| Texas Instruments Incorporated
| CDCLVP1102 1:2 Differential Buffer with one Clock Input
| CDCLVP1204 2:4 Differential Buffer with Selectable Clock Inputs
| CDCLVP1208 Low Jitter 8 Output LVPECL Buffer with Selectable Input
| CDCLVP1212 Low Jitter 12 Output LVPECL Buffer with Selectable Input
| CDCLVP1216 2:16 Differential LVPECL Buffer, High Performance Clock Buffer
| CDCLVP2102 Low Jitter Dual 1:2 LVPECL Buffer
| CDCLVP2104 Low Jitter Dual 1:4 LVPECL Buffer
| CDCLVP2106 Low Jitter Dual 1:6 LVPECL Buffer
| CDCLVP2108 1:8,16 LVPECL Output, no SEL pin,High Performance Clock Buffer
| Marketing part#   Voltage Range   Package-type   #pins/pkg drawing
| CDCLVP1102RGTR   2.375V - 3.6V   QFN   16-pin RGT
| CDCLVP1102RGTT   2.375V - 3.6V   QFN   16-pin RGT
| CDCLVP2102RGTR   2.375V - 3.6V   QFN   16-pin RGT
| CDCLVP2102RGTT   2.375V - 3.6V   QFN   16-pin RGT
| CDCLVP1204RGTR   2.375V - 3.6V   QFN   16-pin RGT
| CDCLVP1204RGTT   2.375V - 3.6V   QFN   16-pin RGT
| CDCLVP1216RGZR   2.375V - 3.6V   QFN   48-pin RGZ
| CDCLVP1216RGZT   2.375V - 3.6V   QFN   48-pin RGZ
| CDCLVP2108RGZR   2.375V - 3.6V   QFN   48-pin RGZ
| CDCLVP2108RGZT   2.375V - 3.6V   QFN   48-pin RGZ
| CDCLVP1212RHAR   2.375V - 3.6V   QFN   40-pin RHA
| CDCLVP1212RHAT   2.375V - 3.6V   QFN   40-pin RHA
| CDCLVP2106RHAR   2.375V - 3.6V   QFN   40-pin RHA
| CDCLVP2106RHAT   2.375V - 3.6V   QFN   40-pin RHA
| CDCLVP1208RHDR   2.375V - 3.6V   QFN   28-pin RHD
| CDCLVP1208RHDT   2.375V - 3.6V   QFN   28-pin RHD
| CDCLVP2104RHDR   2.375V - 3.6V   QFN   28-pin RHD
| CDCLVP2104RHDT   2.375V - 3.6V   QFN   28-pin RHD
[IBIS ver]   4.1
[File name]   cdclvpx.ibs
[File Rev]   1.3
[Date]   09/30/2013
[Source]
| Texas Instruments Incorporated.
| Analog-eLab Design Center, HPA
| 12500 TI Blvd
| Dallas, TX -75243
[Notes]   Revision History
| Rev 1.0: 06/03/2009
| - Initial model generated from Spectre simulations
| - Initial version of the model not matched to
|   measurements
| - Warnings related to VAC_REF clamp characterisitics
|   can be ignored, as they represent true buffer characteristics
| - Initial IBIS file named cdclvp1102.ibs
| Rev 1.1: 07/29/2009
| - File name changed from cdclvp1102.ibs to cdclvpx.ibs
| - Added package models for CDCLVP2102,CDCLVP1204,CDCLVP1216,CDCLVP2108,
|   CDCLVP1212, CDCLVP2106, CDCLVP1208, and CDCLVP2104. All these
|   parts share same set of I/O buffers.
| Rev 1.2: 08/20/2013
| - Added models for 2.5V corner.
| Rev 1.3: 09/30/2013
| - Modified pecl models at 3.3V and 2.5V corners.
|*  EXCEPTION:   *
|*  - For model input_2p5 and sel_in_2p5, there will be a leakage   *
|*   current in the POWER clamp I-V Table because of the transistor   *
|*   XQQ0 connected to the pad.   *
|*  - For model vac_ref_2p5, there will be a leakage current in the   *
|*   GROUND and POWER clamp I-V Table because of the voltage source   *
|*   connected  to the pad.   *
|*  - For model pecl_*, there will be a leakage current in the GROUND   *
|*   clamp I-V Table because of the BJT Q6<1:20>(NPN4T_3V_LC_P25L5)   *
|*   connected to the pad.   *
[Disclaimer]
| This model is designed as an aid for customers of Texas Instruments.
| TI and its licensors and suppliers make no warranties, either expressed
| or implied, with respect to this  model, including the warranties of
| merchantability or fitness for a particular purpose. The model is
| provided solely on an "as is" basis. The entire risk as to its quality
| and performance is with the customer.
[Copyright] (C)Copyright 2013 Texas Instruments Incorporated.
   All rights reserved.
|   Component CDCLVP1102RGT
[Component]   CDCLVP1102RGT
[Manufacturer]  Texas Instruments Incorporated
[Package]   |16-pin QFN RGT package
|   typ   min   max
R_pkg   0.2442   0.2257   0.2626
L_pkg   1.1009nH   1.0046nH   1.1974nH
C_pkg   0.1103pF   0.1081pF   0.1124pF
[Pin] signal_name  model_name   R_pin   L_pin   C_pin
   1   GND   GND   0.12037   0.82216nH   0.12472pF
   2   NC   NC   0.00244   0.06008nH   0.03612pF
   3   NC   NC   0.00244   0.06008nH   0.03612pF
   4   NC   NC   0.00244   0.06216nH   0.03162pF
   5   VCC   POWER   0.12566   0.86112nH   0.13739pF
   6   INP0   INPUT   0.22876   1.02355nH   0.11116pF
   7   INN0   INPUT   0.23258   1.04274nH   0.11153pF
   8   VAC_REF   VAC_REF   0.26260   1.19735nH   0.11242pF
   9   OUTP0   PECL_OUT   0.25027   1.13306nH   0.10811pF
   10   OUTN0   PECL_OUT   0.22571   1.00464nH   0.10867pF
   11   OUTP1   PECL_OUT   0.22940   1.02114nH   0.11008pF
   12   OUTN1   PECL_OUT   0.25984   1.17646nH   0.11074pF
   13   NC   NC   0.00244   0.06216nH   0.03162pF
   14   NC   NC   0.00244   0.06008nH   0.03612pF
   15   NC   NC   0.00244   0.06008nH   0.03612pF
   16   GND   GND   0.12148   0.82689nH   0.12554pF
[Diff_Pin]  inv_pin  vdiff   tdelay_typ  tdelay_min  tdelay_max
| The '+' pin is   Diff_pin,   the '-' pin is the   Inv_pin
| Receiver Pins  |  Receiver Vth = +/-200mV
6   7   0.8V   0ns   0ns   0ns
| LVPECL Driver Pins
9   10   0.5V   0ns   0ns   0ns
11   12   0.5V   0ns   0ns   0ns
|   Component CDCLVP2102RGT
[Component]   CDCLVP2102RGT
[Manufacturer]  Texas Instruments Incorporated
[Package]   |16-pin QFN RGT package
|   typ   min   max
R_pkg   0.2458   0.2257   0.2658
L_pkg   1.1055nH   1.0046nH   1.2064nH
C_pkg   0.1092pF   0.1051pF   0.1132pF
[Pin] signal_name  model_name   R_pin   L_pin   C_pin
   1   GND   GND   0.12037   0.82216nH   0.12819pF
   2   NC   NC   0.00244   0.06008nH   0.03612pF
   3   INP1   INPUT   0.22606   1.00656nH   0.10507pF
   4   INN1   INPUT   0.25236   1.14386nH   0.10913pF
   5   VCC   POWER   0.08325   0.79299nH   0.15518pF
   6   INP0   INPUT   0.22876   1.02355nH   0.11162pF
   7   INN0   INPUT   0.23258   1.04274nH   0.11159pF
   8   VAC_REF   VAC_REF   0.26260   1.19735nH   0.11246pF
   9   OUTP0   PECL_OUT   0.25027   1.13306nH   0.10814pF
   10   OUTN0   PECL_OUT   0.22571   1.00464nH   0.10870pF
   11   OUTP1   PECL_OUT   0.22940   1.02114nH   0.11016pF
   12   OUTN1   PECL_OUT   0.25984   1.17646nH   0.11123pF
   13   OUTP2   PECL_OUT   0.26581   1.20636nH   0.11324pF
   14   OUTN2   PECL_OUT   0.23400   1.04124nH   0.11179pF
   15   OUTP3   PECL_OUT   0.22794   1.01049nH   0.10931pF
   16   OUTN3   PECL_OUT   0.25004   1.12526nH   0.10844pF
[Diff_Pin]  inv_pin  vdiff   tdelay_typ  tdelay_min  tdelay_max
| The '+' pin is   Diff_pin,   the '-' pin is the   Inv_pin
| Receiver Pins  |  Receiver Vth = +/-200mV
3   4   0.8V   0ns   0ns   0ns
6   7   0.8V   0ns   0ns   0ns
| LVPECL Driver Pins
9   10   0.5V   0ns   0ns   0ns
11   12   0.5V   0ns   0ns   0ns
13   14   0.5V   0ns   0ns   0ns
15   16   0.5V   0ns   0ns   0ns
|   Component CDCLVP1204RGT
[Component]   CDCLVP1204RGT
[Manufacturer]  Texas Instruments Incorporated
[Package]   |16-pin QFN RGT package
|   typ   min   max
R_pkg   0.2458   0.2257   0.2658
L_pkg   1.1055nH   1.0046nH   1.2064nH
C_pkg   0.1103pF   0.1073pF   0.1133pF
[Pin] signal_name  model_name   R_pin   L_pin   C_pin
   1   GND   GND   0.12037   0.82216nH   0.12819pF
   2   IN_SEL   SEL_IN   0.22773   1.01285nH   0.10730pF
   3   INP1   INPUT   0.22606   1.00656nH   0.10882pF
   4   INN1   INPUT   0.25236   1.14386nH   0.10955pF
   5   VCC   POWER   0.08325   0.79299nH   0.15524pF
   6   INP0   INPUT   0.22876   1.02355nH   0.11162pF
   7   INN0   INPUT   0.23258   1.04274nH   0.11160pF
   8   VAC_REF   VAC_REF   0.26260   1.19735nH   0.11246pF
   9   OUTP0   PECL_OUT   0.25027   1.13306nH   0.10814pF
   10   OUTN0   PECL_OUT   0.22571   1.00464nH   0.10870pF
   11   OUTP1   PECL_OUT   0.22940   1.02114nH   0.11017pF
   12   OUTN1   PECL_OUT   0.25984   1.17646nH   0.11124pF
   13   OUTP2   PECL_OUT   0.26581   1.20636nH   0.11325pF
   14   OUTN2   PECL_OUT   0.23400   1.04124nH   0.11180pF
   15   OUTP3   PECL_OUT   0.22794   1.01049nH   0.10933pF
   16   OUTN3   PECL_OUT   0.25004   1.12526nH   0.10849pF
[Diff_Pin]  inv_pin  vdiff   tdelay_typ  tdelay_min  tdelay_max
| The '+' pin is   Diff_pin,   the '-' pin is the   Inv_pin
| Receiver Pins  |  Receiver Vth = +/-200mV
3   4   0.8V   0ns   0ns   0ns
6   7   0.8V   0ns   0ns   0ns
| LVPECL Driver Pins
9   10   0.5V   0ns   0ns   0ns
11   12   0.5V   0ns   0ns   0ns
13   14   0.5V   0ns   0ns   0ns
15   16   0.5V   0ns   0ns   0ns
[series pin mapping]  pin_2   model_name
2   1   pdn_sel_in
|   Component CDCLVP1216RGZ
[Component]   CDCLVP1216RGZ
[Manufacturer]  Texas Instruments Incorporated
[Package]   |48-pin QFN RGZ, 7mm X 7mm package
|   typ   min   max
R_pkg   0.588   0.510   0.665
L_pkg   2.957nH   2.542nH   3.371nH
C_pkg   0.272pF   0.247pF   0.297pF
[Pin] signal_name  model_name   R_pin   L_pin   C_pin
   1   GND   GND   0.65656   3.33539nH   0.28003pF
   2   IN_SEL   SEL_IN   0.61157   3.08921nH   0.28915pF
   3   INP1   INPUT   0.57343   2.88428nH   0.27264pF
   4   INN1   INPUT   0.54341   2.72363nH   0.25062pF
   5   NC   NC   0.00473   0.11459nH   0.07856pF
   6   VCC   POWER   0.25969   2.00218nH   0.30564pF
   7   VCC   POWER   0.51372   2.56508nH   0.24941pF
   8   VAC_REF   VAC_REF   0.52312   2.61529nH   0.25165pF
   9   INN0   INPUT   0.54343   2.72383nH   0.25978pF
   10   INP0   INPUT   0.57346   2.88448nH   0.26061pF
   11   NC   NC   0.00473   0.11551nH   0.07850pF
   12   GND   GND   0.65660   3.33559nH   0.26143pF
   13   VCC   POWER   0.65496   3.32619nH   0.27810pF
   14   OUTP0   PECL_OUT   0.61059   3.08261nH   0.28822pF
   15   OUTN0   PECL_OUT   0.57193   2.87407nH   0.27296pF
   16   OUTP1   PECL_OUT   0.54137   2.70952nH   0.26007pF
   17   OUTN1   PECL_OUT   0.52043   2.59668nH   0.25132pF
   18   OUTP2   PECL_OUT   0.51043   2.54238nH   0.24716pF
   19   OUTN2   PECL_OUT   0.51205   2.55018nH   0.24780pF
   20   OUTP3   PECL_OUT   0.52519   2.61949nH   0.25320pF
   21   OUTN3   PECL_OUT   0.54894   2.74573nH   0.26313pF
   22   OUTP4   PECL_OUT   0.58191   2.92178nH   0.27726pF
   23   OUTN4   PECL_OUT   0.62252   3.13971nH   0.29741pF
   24   VCC   POWER   0.33317   2.81171nH   0.35197pF
   25   OUTP5   PECL_OUT   0.66500   3.37178nH   0.28261pF
   26   OUTN5   PECL_OUT   0.61921   3.12071nH   0.29202pF
   27   OUTP6   PECL_OUT   0.57979   2.90827nH   0.27574pF
   28   OUTN6   PECL_OUT   0.54821   2.73883nH   0.26237pF
   29   OUTP7   PECL_OUT   0.52603   2.61989nH   0.25309pF
   30   OUTN7   PECL_OUT   0.51455   2.55838nH   0.24823pF
   31   OUTP8   PECL_OUT   0.51455   2.55838nH   0.24822pF
   32   OUTN8   PECL_OUT   0.52601   2.61979nH   0.25309pF
   33   OUTP9   PECL_OUT   0.54819   2.73873nH   0.26236pF
   34   OUTN9   PECL_OUT   0.57976   2.90818nH   0.27572pF
   35   OUTP10   PECL_OUT   0.61918   3.12051nH   0.29200pF
   36   OUTN10   PECL_OUT   0.66496   3.37159nH   0.28258pF
   37   VCC   POWER   0.33314   2.82774nH   0.35201pF
   38   OUTP11   PECL_OUT   0.62248   3.13941nH   0.29741pF
   39   OUTN11   PECL_OUT   0.58186   2.92147nH   0.27725pF
   40   OUTP12   PECL_OUT   0.54889   2.74553nH   0.26312pF
   41   OUTN12   PECL_OUT   0.52513   2.61919nH   0.25318pF
   42   OUTP13   PECL_OUT   0.51200   2.54988nH   0.24778pF
   43   OUTN13   PECL_OUT   0.51036   2.54206nH   0.24716pF
   44   OUTP14   PECL_OUT   0.52038   2.59649nH   0.25131pF
   45   OUTN14   PECL_OUT   0.54131   2.70921nH   0.26007pF
   46   OUTP15   PECL_OUT   0.57189   2.87377nH   0.27298pF
   47   OUTN15   PECL_OUT   0.61053   3.08229nH   0.28833pF
   48   VCC   POWER   0.65491   3.32598nH   0.27862pF
[Diff_Pin]  inv_pin  vdiff   tdelay_typ  tdelay_min  tdelay_max
| The '+' pin is   Diff_pin,   the '-' pin is the   Inv_pin
| Receiver Pins  |  Receiver Vth = +/-200mV
3   4   0.8V   0ns   0ns   0ns
9   10   0.8V   0ns   0ns   0ns
| LVPECL Driver Pins
14   15   0.5V   0ns   0ns   0ns
16   17   0.5V   0ns   0ns   0ns
18   19   0.5V   0ns   0ns   0ns
20   21   0.5V   0ns   0ns   0ns
22   23   0.5V   0ns   0ns   0ns
25   26   0.5V   0ns   0ns   0ns
27   28   0.5V   0ns   0ns   0ns
29   30   0.5V   0ns   0ns   0ns
31   32   0.5V   0ns   0ns   0ns
33   34   0.5V   0ns   0ns   0ns
35   36   0.5V   0ns   0ns   0ns
38   39   0.5V   0ns   0ns   0ns
40   41   0.5V   0ns   0ns   0ns
42   43   0.5V   0ns   0ns   0ns
44   45   0.5V   0ns   0ns   0ns
46   47   0.5V   0ns   0ns   0ns
[series pin mapping]  pin_2   model_name
2   1   pdn_sel_in
|   Component CDCLVP1216RGZ
[Component]   CDCLVP2108RGZ
[Manufacturer]  Texas Instruments Incorporated
[Package]   |48-pin QFN RGZ, 7mm X 7mm package
|   typ   min   max
R_pkg   0.588   0.510   0.665
L_pkg   2.957nH   2.542nH   3.371nH
C_pkg   0.272pF   0.247pF   0.297pF
[Pin] signal_name  model_name   R_pin   L_pin   C_pin
   1   GND   GND   0.65656   3.33539nH   0.28003pF
   2   NC   NC   0.00473   0.11551nH   0.07850pF
   3   INP1   INPUT   0.57343   2.88428nH   0.27264pF
   4   INN1   INPUT   0.54341   2.72363nH   0.25062pF
   5   VAC_REF1   VAC_REF   0.52311   2.61519nH   0.25495pF
   6   VCC   POWER   0.25969   2.00218nH   0.30564pF
   7   VCC   POWER   0.51372   2.56508nH   0.24941pF
   8   VAC_REF0   VAC_REF   0.52312   2.61529nH   0.25165pF
   9   INN0   INPUT   0.54343   2.72383nH   0.25978pF
   10   INP0   INPUT   0.57346   2.88448nH   0.26061pF
   11   NC   NC   0.00473   0.11551nH   0.07850pF
   12   GND   GND   0.65660   3.33559nH   0.26143pF
   13   VCC   POWER   0.65496   3.32619nH   0.27810pF
   14   OUTP0   PECL_OUT   0.61059   3.08261nH   0.28822pF
   15   OUTN0   PECL_OUT   0.57193   2.87407nH   0.27296pF
   16   OUTP1   PECL_OUT   0.54137   2.70952nH   0.26007pF
   17   OUTN1   PECL_OUT   0.52043   2.59668nH   0.25132pF
   18   OUTP2   PECL_OUT   0.51043   2.54238nH   0.24716pF
   19   OUTN2   PECL_OUT   0.51205   2.55018nH   0.24780pF
   20   OUTP3   PECL_OUT   0.52519   2.61949nH   0.25320pF
   21   OUTN3   PECL_OUT   0.54894   2.74573nH   0.26313pF
   22   OUTP4   PECL_OUT   0.58191   2.92178nH   0.27726pF
   23   OUTN4   PECL_OUT   0.62252   3.13971nH   0.29741pF
   24   VCC   POWER   0.33317   2.81171nH   0.35197pF
   25   OUTP5   PECL_OUT   0.66500   3.37178nH   0.28261pF
   26   OUTN5   PECL_OUT   0.61921   3.12071nH   0.29202pF
   27   OUTP6   PECL_OUT   0.57979   2.90827nH   0.27574pF
   28   OUTN6   PECL_OUT   0.54821   2.73883nH   0.26237pF
   29   OUTP7   PECL_OUT   0.52603   2.61989nH   0.25309pF
   30   OUTN7   PECL_OUT   0.51455   2.55838nH   0.24823pF
   31   OUTP8   PECL_OUT   0.51455   2.55838nH   0.24822pF
   32   OUTN8   PECL_OUT   0.52601   2.61979nH   0.25309pF
   33   OUTP9   PECL_OUT   0.54819   2.73873nH   0.26236pF
   34   OUTN9   PECL_OUT   0.57976   2.90818nH   0.27572pF
   35   OUTP10   PECL_OUT   0.61918   3.12051nH   0.29200pF
   36   OUTN10   PECL_OUT   0.66496   3.37159nH   0.28258pF
   37   VCC   POWER   0.33314   2.82774nH   0.35201pF
   38   OUTP11   PECL_OUT   0.62248   3.13941nH   0.29741pF
   39   OUTN11   PECL_OUT   0.58186   2.92147nH   0.27725pF
   40   OUTP12   PECL_OUT   0.54889   2.74553nH   0.26312pF
   41   OUTN12   PECL_OUT   0.52513   2.61919nH   0.25318pF
   42   OUTP13   PECL_OUT   0.51200   2.54988nH   0.24778pF
   43   OUTN13   PECL_OUT   0.51036   2.54206nH   0.24716pF
   44   OUTP14   PECL_OUT   0.52038   2.59649nH   0.25131pF
   45   OUTN14   PECL_OUT   0.54131   2.70921nH   0.26007pF
   46   OUTP15   PECL_OUT   0.57189   2.87377nH   0.27298pF
   47   OUTN15   PECL_OUT   0.61053   3.08229nH   0.28833pF
   48   VCC   POWER   0.65491   3.32598nH   0.27862pF
[Diff_Pin]  inv_pin  vdiff   tdelay_typ  tdelay_min  tdelay_max
| The '+' pin is   Diff_pin,   the '-' pin is the   Inv_pin
| Receiver Pins  |  Receiver Vth = +/-200mV
3   4   0.8V   0ns   0ns   0ns
9   10   0.8V   0ns   0ns   0ns
| LVPECL Driver Pins
14   15   0.5V   0ns   0ns   0ns
16   17   0.5V   0ns   0ns   0ns
18   19   0.5V   0ns   0ns   0ns
20   21   0.5V   0ns   0ns   0ns
22   23   0.5V   0ns   0ns   0ns
25   26   0.5V   0ns   0ns   0ns
27   28   0.5V   0ns   0ns   0ns
29   30   0.5V   0ns   0ns   0ns
31   32   0.5V   0ns   0ns   0ns
33   34   0.5V   0ns   0ns   0ns
35   36   0.5V   0ns   0ns   0ns
38   39   0.5V   0ns   0ns   0ns
40   41   0.5V   0ns   0ns   0ns
42   43   0.5V   0ns   0ns   0ns
44   45   0.5V   0ns   0ns   0ns
46   47   0.5V   0ns   0ns   0ns
|   Component CDCLVP1212RHA
[Component]   CDCLVP1212RHA
[Manufacturer]  Texas Instruments Incorporated
[Package]   |40-pin QFN RHA, 6mm X 6mm package
|   typ   min   max
R_pkg   0.479   0.421   0.537
L_pkg   2.328nH   2.014nH   2.641nH
C_pkg   0.205pF   0.184pF   0.226pF
[Pin] signal_name  model_name   R_pin   L_pin   C_pin
   1   IN_SEL   SEL_IN   0.53663   2.64121nH   0.21428pF
   2   INP1   INPUT   0.49495   2.41562nH   0.22153pF
   3   INN1   INPUT   0.45957   2.22655nH   0.19938pF
   4   NC   NC   0.00171   0.04929nH   0.05222pF
   5   VCC   POWER   0.21322   1.56144nH   0.24182pF
   6   VCC   POWER   0.42364   2.03554nH   0.19378pF
   7   VAC_REF   VAC_REF   0.43514   2.09659nH   0.19724pF
   8   INN0   INPUT   0.45959   2.22665nH   0.20687pF
   9   INP0   INPUT   0.49499   2.41572nH   0.20752pF
   10   NC   NC   0.00171   0.05331nH   0.04134pF
   11   VCC   POWER   0.52466   2.57661nH   0.19722pF
   12   OUTP0   PECL_OUT   0.50327   2.45872nH   0.21745pF
   13   OUTN0   PECL_OUT   0.46514   2.25385nH   0.20998pF
   14   OUTP1   PECL_OUT   0.43728   2.10459nH   0.19877pF
   15   OUTN1   PECL_OUT   0.42197   2.02214nH   0.19250pF
   16   OUTP2   PECL_OUT   0.42072   2.01434nH   0.19197pF
   17   OUTN2   PECL_OUT   0.43367   2.08219nH   0.19731pF
   18   OUTP3   PECL_OUT   0.45950   2.21885nH   0.20822pF
   19   OUTN3   PECL_OUT   0.49602   2.41352nH   0.22636pF
   20   VCC   POWER   0.26646   2.10219nH   0.28000pF
   21   GND   GND   0.52445   2.56751nH   0.21245pF
   22   OUTP4   PECL_OUT   0.48448   2.35042nH   0.21789pF
   23   OUTN4   PECL_OUT   0.45183   2.17535nH   0.20432pF
   24   OUTP5   PECL_OUT   0.43066   2.06239nH   0.19495pF
   25   OUTN5   PECL_OUT   0.42289   2.02094nH   0.18444pF
   26   OUTP6   PECL_OUT   0.42289   2.02094nH   0.18443pF
   27   OUTN6   PECL_OUT   0.43065   2.06229nH   0.19494pF
   28   OUTP7   PECL_OUT   0.45180   2.17525nH   0.20432pF
   29   OUTN7   PECL_OUT   0.48445   2.35022nH   0.21788pF
   30   GND   GND   0.52441   2.56731nH   0.21245pF
   31   VCC   POWER   0.26643   2.10828nH   0.28002pF
   32   OUTP8   PECL_OUT   0.49598   2.41332nH   0.22636pF
   33   OUTN8   PECL_OUT   0.45945   2.21865nH   0.20820pF
   34   OUTP9   PECL_OUT   0.43362   2.08189nH   0.19730pF
   35   OUTN9   PECL_OUT   0.42067   2.01414nH   0.19196pF
   36   OUTP10   PECL_OUT   0.42192   2.02184nH   0.19248pF
   37   OUTN10   PECL_OUT   0.43723   2.10429nH   0.19877pF
   38   OUTP11   PECL_OUT   0.46509   2.25365nH   0.21002pF
   39   OUTN11   PECL_OUT   0.50323   2.45852nH   0.21772pF
   40   VCC   POWER   0.52461   2.57631nH   0.20060pF
[Diff_Pin]  inv_pin  vdiff   tdelay_typ  tdelay_min  tdelay_max
| The '+' pin is   Diff_pin,   the '-' pin is the   Inv_pin
| Receiver Pins  |  Receiver Vth = +/-200mV
2   3   0.8V   0ns   0ns   0ns
8   9   0.8V   0ns   0ns   0ns
| LVPECL Driver Pins
12   13   0.5V   0ns   0ns   0ns
14   15   0.5V   0ns   0ns   0ns
16   17   0.5V   0ns   0ns   0ns
18   19   0.5V   0ns   0ns   0ns
22   23   0.5V   0ns   0ns   0ns
24   25   0.5V   0ns   0ns   0ns
26   27   0.5V   0ns   0ns   0ns
28   29   0.5V   0ns   0ns   0ns
32   33   0.5V   0ns   0ns   0ns
34   35   0.5V   0ns   0ns   0ns
36   37   0.5V   0ns   0ns   0ns
38   39   0.5V   0ns   0ns   0ns
[series pin mapping]  pin_2   model_name
1   21   pdn_sel_in
|   Component CDCLVP2106RHA
[Component]   CDCLVP2106RHA
[Manufacturer]  Texas Instruments Incorporated
[Package]   |40-pin QFN RHA, 6mm X 6mm package
|   typ   min   max
R_pkg   0.462   0.421   0.503
L_pkg   2.326nH   2.014nH   2.659nH
C_pkg   0.205pF   0.184pF   0.226pF
[Pin] signal_name  model_name   R_pin   L_pin   C_pin
   1   NC   NC   0.00171   0.05331nH   0.04133pF
   2   INP1   INPUT   0.49495   2.41562nH   0.22153pF
   3   INN1   INPUT   0.45957   2.22655nH   0.19938pF
   4   VAC_REF1   VAC_REF   0.43512   2.09649nH   0.19991pF
   5   VCC   POWER   0.21322   1.56144nH   0.24182pF
   6   VCC   POWER   0.42364   2.03554nH   0.19378pF
   7   VAC_REF0   VAC_REF   0.43514   2.09659nH   0.19724pF
   8   INN0   INPUT   0.45959   2.22665nH   0.20687pF
   9   INP0   INPUT   0.49499   2.41572nH   0.20752pF
   10   NC   NC   0.00171   0.05331nH   0.04134pF
   11   VCC   POWER   0.52466   2.57661nH   0.19722pF
   12   OUTP0   PECL_OUT   0.50327   2.45872nH   0.21745pF
   13   OUTN0   PECL_OUT   0.46514   2.25385nH   0.20998pF
   14   OUTP1   PECL_OUT   0.43728   2.10459nH   0.19877pF
   15   OUTN1   PECL_OUT   0.42197   2.02214nH   0.19250pF
   16   OUTP2   PECL_OUT   0.42072   2.01434nH   0.19197pF
   17   OUTN2   PECL_OUT   0.43367   2.08219nH   0.19731pF
   18   OUTP3   PECL_OUT   0.45950   2.21885nH   0.20822pF
   19   OUTN3   PECL_OUT   0.49602   2.41352nH   0.22636pF
   20   VCC   POWER   0.26646   2.10219nH   0.28000pF
   21   GND   GND   0.52445   2.56751nH   0.21245pF
   22   OUTP4   PECL_OUT   0.48448   2.35042nH   0.21789pF
   23   OUTN4   PECL_OUT   0.45183   2.17535nH   0.20432pF
   24   OUTP5   PECL_OUT   0.43066   2.06239nH   0.19495pF
   25   OUTN5   PECL_OUT   0.42289   2.02094nH   0.18444pF
   26   OUTP6   PECL_OUT   0.42289   2.02094nH   0.18443pF
   27   OUTN6   PECL_OUT   0.43065   2.06229nH   0.19494pF
   28   OUTP7   PECL_OUT   0.45180   2.17525nH   0.20432pF
   29   OUTN7   PECL_OUT   0.48445   2.35022nH   0.21788pF
   30   GND   GND   0.52441   2.56731nH   0.21245pF
   31   VCC   POWER   0.26643   2.10828nH   0.28002pF
   32   OUTP8   PECL_OUT   0.49598   2.41332nH   0.22636pF
   33   OUTN8   PECL_OUT   0.45945   2.21865nH   0.20820pF
   34   OUTP9   PECL_OUT   0.43362   2.08189nH   0.19730pF
   35   OUTN9   PECL_OUT   0.42067   2.01414nH   0.19196pF
   36   OUTP10   PECL_OUT   0.42192   2.02184nH   0.19248pF
   37   OUTN10   PECL_OUT   0.43723   2.10429nH   0.19877pF
   38   OUTP11   PECL_OUT   0.46509   2.25365nH   0.21002pF
   39   OUTN11   PECL_OUT   0.50323   2.45852nH   0.21772pF
   40   VCC   POWER   0.52461   2.57631nH   0.20060pF
[Diff_Pin]  inv_pin  vdiff   tdelay_typ  tdelay_min  tdelay_max
| The '+' pin is   Diff_pin,   the '-' pin is the   Inv_pin
| Receiver Pins  |  Receiver Vth = +/-200mV
2   3   0.8V   0ns   0ns   0ns
8   9   0.8V   0ns   0ns   0ns
| LVPECL Driver Pins
12   13   0.5V   0ns   0ns   0ns
14   15   0.5V   0ns   0ns   0ns
16   17   0.5V   0ns   0ns   0ns
18   19   0.5V   0ns   0ns   0ns
22   23   0.5V   0ns   0ns   0ns
24   25   0.5V   0ns   0ns   0ns
26   27   0.5V   0ns   0ns   0ns
28   29   0.5V   0ns   0ns   0ns
32   33   0.5V   0ns   0ns   0ns
34   35   0.5V   0ns   0ns   0ns
36   37   0.5V   0ns   0ns   0ns
38   39   0.5V   0ns   0ns   0ns
|   Component CDCLVP1208RHD
[Component]   CDCLVP1208RHD
[Manufacturer]  Texas Instruments Incorporated
[Package]   |28-pin QFN RHD, 5mm X 5mm package
|   typ   min   max
R_pkg   0.376   0.336   0.416
L_pkg   1.773nH   1.560nH   1.986nH
C_pkg   0.184pF   0.173pF   0.196pF
[Pin] signal_name  model_name   R_pin   L_pin   C_pin
   1   GND   GND   0.20205   1.54413nH   0.22779pF
   2   OUTP7   PECL_OUT   0.36833   1.73054nH   0.19140pF
   3   OUTN7   PECL_OUT   0.34356   1.60090nH   0.17840pF
   4   IN_SEL   SEL_IN   0.33554   1.56003nH   0.17503pF
   5   INP1   INPUT   0.34557   1.61410nH   0.17912pF
   6   INN1   INPUT   0.37204   1.75504nH   0.18953pF
   7   VAC_REF   VAC_REF   0.41113   1.96558nH   0.17941pF
   8   VCC   POWER   0.20608   1.47220nH   0.23933pF
   9   INP0   INPUT   0.38079   1.80314nH   0.19569pF
   10   INN0   INPUT   0.35247   1.65370nH   0.17560pF
   11   NC   NC   0.00139   0.04443nH   0.06337pF
   12   OUTP0   PECL_OUT   0.34512   1.61530nH   0.17275pF
   13   OUTN0   PECL_OUT   0.36718   1.73174nH   0.18738pF
   14   GND   GND   0.40372   1.92738nH   0.17766pF
   15   VCC   POWER   0.20323   1.55915nH   0.22711pF
   16   OUTP1   PECL_OUT   0.37026   1.74564nH   0.19232pF
   17   OUTN1   PECL_OUT   0.34486   1.61030nH   0.17896pF
   18   OUTP2   PECL_OUT   0.33606   1.56273nH   0.17520pF
   19   OUTN2   PECL_OUT   0.34529   1.60990nH   0.17885pF
   20   OUTP3   PECL_OUT   0.37105   1.74484nH   0.18893pF
   21   OUTN3   PECL_OUT   0.40991   1.95238nH   0.17780pF
   22   OUTP4   PECL_OUT   0.41637   1.98558nH   0.17997pF
   23   OUTN4   PECL_OUT   0.37690   1.77334nH   0.19100pF
   24   OUTP5   PECL_OUT   0.35016   1.63170nH   0.18046pF
   25   OUTN5   PECL_OUT   0.33957   1.57583nH   0.17618pF
   26   OUTP6   PECL_OUT   0.34680   1.61400nH   0.17927pF
   27   OUTN6   PECL_OUT   0.37068   1.74054nH   0.19195pF
   28   VCC   POWER   0.20285   1.53973nH   0.22849pF
[Diff_Pin]  inv_pin  vdiff   tdelay_typ  tdelay_min  tdelay_max
| The '+' pin is   Diff_pin,   the '-' pin is the   Inv_pin
| Receiver Pins  |  Receiver Vth = +/-200mV
5   6   0.8V   0ns   0ns   0ns
9   10   0.8V   0ns   0ns   0ns
| LVPECL Driver Pins
2   3   0.5V   0ns   0ns   0ns
12   13   0.5V   0ns   0ns   0ns
16   17   0.5V   0ns   0ns   0ns
18   19   0.5V   0ns   0ns   0ns
20   21   0.5V   0ns   0ns   0ns
22   23   0.5V   0ns   0ns   0ns
24   25   0.5V   0ns   0ns   0ns
26   27   0.5V   0ns   0ns   0ns
[series pin mapping]  pin_2   model_name
4   1   pdn_sel_in
|   Component CDCLVP2104RHD
[Component]   CDCLVP2104RHD
[Manufacturer]  Texas Instruments Incorporated
[Package]   |28-pin QFN RHD, 5mm X 5mm package
|   typ   min   max
R_pkg   0.376   0.336   0.416
L_pkg   1.773nH   1.560nH   1.986nH
C_pkg   0.184pF   0.173pF   0.196pF
[Pin] signal_name  model_name   R_pin   L_pin   C_pin
   1   GND   GND   0.20205   1.54413nH   0.22779pF
   2   OUTP7   PECL_OUT   0.36833   1.73054nH   0.19140pF
   3   OUTN7   PECL_OUT   0.34356   1.60090nH   0.17840pF
   4   NC   NC   0.00139   0.04443nH   0.06337pF
   5   INP1   INPUT   0.34557   1.61410nH   0.17912pF
   6   INN1   INPUT   0.37204   1.75504nH   0.18953pF
   7   VAC_REF1   VAC_REF   0.41113   1.96558nH   0.17941pF
   8   VCC   POWER   0.20608   1.47220nH   0.23933pF
   9   INP0   INPUT   0.38079   1.80314nH   0.19569pF
   10   INN0   INPUT   0.35247   1.65370nH   0.17560pF
   11   VAC_REF0   VAC_REF   0.00139   0.04443nH   0.06337pF
   12   OUTP0   PECL_OUT   0.34512   1.61530nH   0.17275pF
   13   OUTN0   PECL_OUT   0.36718   1.73174nH   0.18738pF
   14   GND   GND   0.40372   1.92738nH   0.17766pF
   15   VCC   POWER   0.20323   1.55915nH   0.22711pF
   16   OUTP1   PECL_OUT   0.37026   1.74564nH   0.19232pF
   17   OUTN1   PECL_OUT   0.34486   1.61030nH   0.17896pF
   18   OUTP2   PECL_OUT   0.33606   1.56273nH   0.17520pF
   19   OUTN2   PECL_OUT   0.34529   1.60990nH   0.17885pF
   20   OUTP3   PECL_OUT   0.37105   1.74484nH   0.18893pF
   21   OUTN3   PECL_OUT   0.40991   1.95238nH   0.17780pF
   22   OUTP4   PECL_OUT   0.41637   1.98558nH   0.17997pF
   23   OUTN4   PECL_OUT   0.37690   1.77334nH   0.19100pF
   24   OUTP5   PECL_OUT   0.35016   1.63170nH   0.18046pF
   25   OUTN5   PECL_OUT   0.33957   1.57583nH   0.17618pF
   26   OUTP6   PECL_OUT   0.34680   1.61400nH   0.17927pF
   27   OUTN6   PECL_OUT   0.37068   1.74054nH   0.19195pF
   28   VCC   POWER   0.20285   1.53973nH   0.22849pF
[Diff_Pin]  inv_pin  vdiff   tdelay_typ  tdelay_min  tdelay_max
| The '+' pin is   Diff_pin,   the '-' pin is the   Inv_pin
| Receiver Pins  |  Receiver Vth = +/-200mV
5   6   0.8V   0ns   0ns   0ns
9   10   0.8V   0ns   0ns   0ns
| LVPECL Driver Pins
2   3   0.5V   0ns   0ns   0ns
12   13   0.5V   0ns   0ns   0ns
16   17   0.5V   0ns   0ns   0ns
18   19   0.5V   0ns   0ns   0ns
20   21   0.5V   0ns   0ns   0ns
22   23   0.5V   0ns   0ns   0ns
24   25   0.5V   0ns   0ns   0ns
26   27   0.5V   0ns   0ns   0ns
|   Model Selectors
[Model Selector] INPUT
input_3p3  3.3V digital input
input_2p5  2.5V digital input
[Model Selector] SEL_IN
sel_in_3p3  3.3V digital input
sel_in_2p5  2.5V digital input
[Model Selector] VAC_REF
vac_ref_3p3  3.3V terminator
vac_ref_2p5  2.5V terminator
[Model Selector] PECL_OUT
pecl_3p3   3.3V digital open_source
pecl_2p5   2.5V digital open_source
| Pulldown resistor on Sel_in, series model of 150kOhm to GND
[Model]   pdn_sel_in
Model_type   Series
C_comp   0pF   0pF   0pF
| Where nom  PVT is Nominal Process, 3.3V, 40C
|   Fast PVT is Strong Process,  3.6V, -40C
|   Slow PVT is Weak Process,   2.375V,100C
[Voltage Range]   3.3V   2.375V   3.6V
[Pullup Reference]   3.3V   2.375V   3.6V
| Junction Temperature (Ambient temp is 25C typ, 85C min, -40C max)
[Temperature Range]   40.0   100.0   -40.0
[R series]   150000   150000   150000
| Models and submodels in the file (9): pdn_sel_in (Series), vac_ref_3p3 (Terminator), vac_ref_2p5 (Terminator), input_3p3 (Input), input_2p5 (Input), sel_in_3p3 (Input), sel_in_2p5 (Input), pecl_3p3 (Open_source), pecl_2p5 (Open_source)
